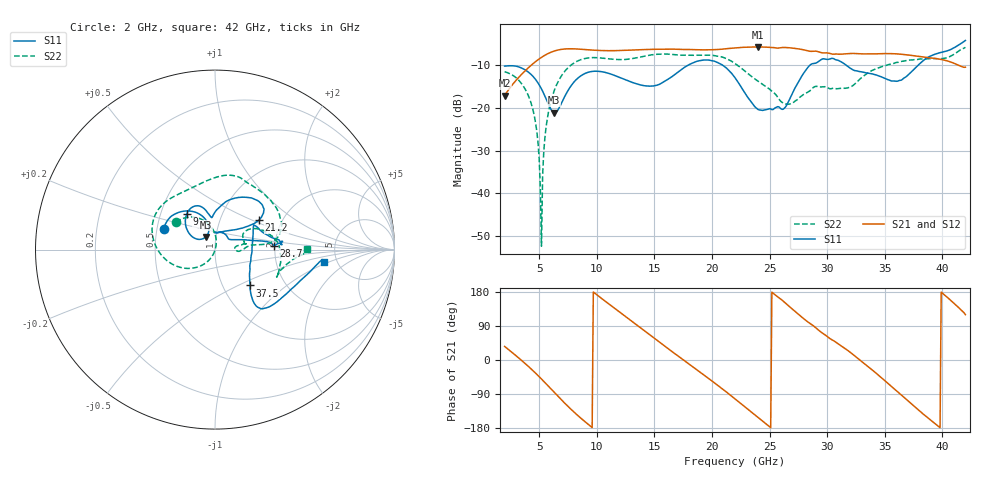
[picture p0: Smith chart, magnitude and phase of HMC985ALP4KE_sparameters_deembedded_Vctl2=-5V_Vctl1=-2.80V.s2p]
!s2p File: Measurements: S11, S21, S12, S22
# GHz S dB R 50.0
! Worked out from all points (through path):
!   401 points, 2 GHz to 42 GHz, reference 50 ohm
!   highest |S21| = -5.76 dB at 24 GHz (marker M1); lowest = -17.1 dB at 2 GHz (marker M2)
!   lowest |S11| = -21.2 dB at 6.3 GHz (marker M3), VSWR 1.19, Z = 44.6 + j6.3 ohm
!   |S11| at or under -10 dB: start of sweep to 17.94 GHz; 20.92 GHz to 28.51 GHz (7.598 GHz wide, 30.7 % of centre); 31.64 GHz to 37.91 GHz (6.272 GHz wide, 18 % of centre)
!   |S22| runs from -52.4 to -5.8 dB; largest |S21 - S12| = 0.0006
!   S11 on the Smith chart (normalised r, x): 2 GHz: 0.54, +0.14; 9 GHz: 0.68, +0.29; 21.2 GHz: 1.53, +0.55; 28.7 GHz: 1.97, +0.10; 37.5 GHz: 1.34, -0.58; 42 GHz: 3.97, -0.88
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2  -10.24 158.1  -17.13 35.8  -17.14 35.8  -11.54 145.2
4.2  -11.94 122.1  -10.29 -20.7  -10.29 -20.7  -18.11 98.6
4.7  -13.41 113.3  -9.16 -35.0  -9.16 -35.0  -23.70 85.2
5  -14.61 108.7  -8.56 -44.0  -8.56 -44.0  -31.89 76.1
5.2  -15.58 106.4  -8.19 -50.2  -8.19 -50.1  -52.35 -87.2
5.7  -18.49 106.3  -7.40 -65.9  -7.40 -65.9  -22.63 -121.1
6.3  -21.16 126.7  -6.72 -85.1  -6.72 -85.1  -16.04 -139.5
8.7  -12.37 132.8  -6.31 -155.6  -6.31 -155.6  -8.66 161.7
9  -11.93 128.5  -6.37 -163.3  -6.38 -163.3  -8.44 156.4
12.6  -13.57 101.4  -6.54 112.5  -6.55 112.5  -8.66 108.3
15.4  -14.54 93.8  -6.29 48.2  -6.29 48.2  -7.44 76.8
18.1  -9.78 64.0  -6.36 -12.8  -6.36 -12.8  -7.70 56.3
21.2  -10.57 33.8  -6.18 -83.1  -6.19 -83.1  -8.45 15.4
22  -12.94 35.4  -5.97 -102.6  -5.98 -102.6  -9.62 8.4
24  -20.38 80.2  -5.76 -151.4  -5.76 -151.4  -13.80 7.0
26.3  -20.05 34.8  -5.88 152.2  -5.88 152.2  -19.01 0.6
28.7  -9.68 3.8  -6.78 92.7  -6.78 92.7  -15.47 11.2
32.4  -11.29 23.7  -7.29 10.6  -7.29 10.7  -14.41 30.8
35.4  -13.52 7.9  -7.31 -65.0  -7.31 -65.0  -9.87 14.3
37.5  -11.09 -45.7  -7.79 -120.9  -7.79 -120.9  -8.77 -3.8
39.7  -7.16 -46.9  -8.58 -176.1  -8.58 -176.1  -8.51 -23.8
42  -4.24 -6.5  -10.50 119.8  -10.51 119.8  -5.84 0.2
